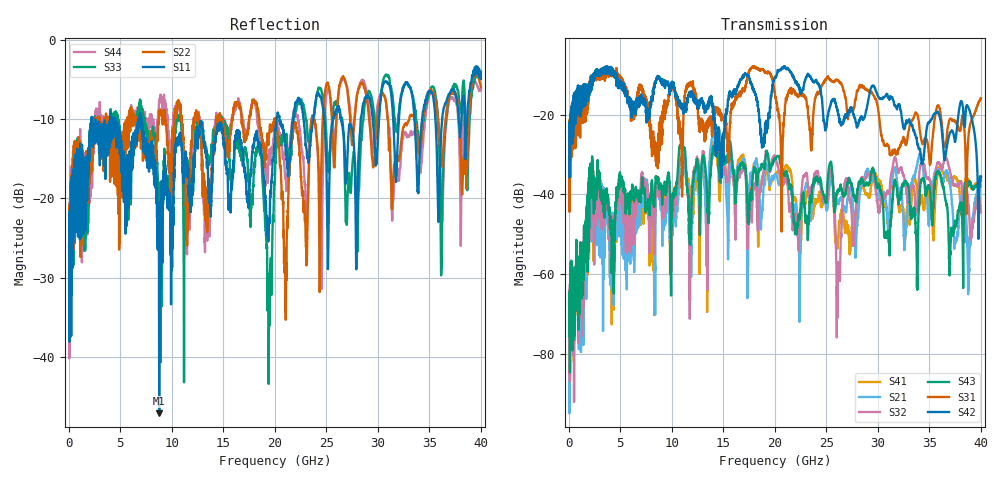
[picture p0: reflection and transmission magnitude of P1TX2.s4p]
!Agilent Technologies,N5245A,MY49151084,A.09.20.08
!Agilent N5245A: A.09.20.08
!Date: Thursday, March 01, 2012 13:18:28
!Correction: S11(Full 4 Port(1,2,3,4))
!S12(Full 4 Port(1,2,3,4))
!S13(Full 4 Port(1,2,3,4))
!S14(Full 4 Port(1,2,3,4))
!S21(Full 4 Port(1,2,3,4))
!S22(Full 4 Port(1,2,3,4))
!S23(Full 4 Port(1,2,3,4))
!S24(Full 4 Port(1,2,3,4))
!S31(Full 4 Port(1,2,3,4))
!S32(Full 4 Port(1,2,3,4))
!S33(Full 4 Port(1,2,3,4))
!S34(Full 4 Port(1,2,3,4))
!S41(Full 4 Port(1,2,3,4))
!S42(Full 4 Port(1,2,3,4))
!S43(Full 4 Port(1,2,3,4))
!S44(Full 4 Port(1,2,3,4))
!S4P File: Measurements: <S11,S12,S13,S14>,
!<S21,S22,S23,S24>,
!<S31,S32,S33,S34>,
!<S41,S42,S43,S44>:
# Hz S  dB  R 50
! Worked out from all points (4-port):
!   3996 points, 50 MHz to 40 GHz, reference 50 ohm
!   strongest paths, dB at 50 MHz, 10.04 GHz, 20.03 GHz, 30.02 GHz, 40 GHz:
!     S42: -24.5, -12.6, -10.8, -15.4, -35.8
!     S31: -25.5, -12.9, -15.1, -18.3, -15.9
!     S43: -67.0, -44.3, -31.1, -37.6, -36.4
!     S32: -64.1, -48.6, -30.6, -43.5, -44.5
!     S21: -69.5, -48.2, -35.1, -38.4, -37.9
!     S41: -64.8, -41.7, -35.2, -36.3, -35.7
!   lowest |S11| = -47.1 dB at 8.79 GHz (marker M1), VSWR 1.01, Z = 49.7 + j0.265 ohm
!   |S11| at or under -10 dB: start of sweep to 2.234 GHz; 4.58 GHz to 6.79 GHz (2.21 GHz wide, 38.9 % of centre); 7.032 GHz to 20.17 GHz (13.13 GHz wide, 96.6 % of centre)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
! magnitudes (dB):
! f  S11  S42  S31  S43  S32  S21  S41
! 50 MHz  -24.1  -24.5  -25.5  -67.0  -64.1  -69.5  -64.8
! 2.18 GHz  -11.9  -11.5  -10.8  -40.8  -45.9  -42.2  -39.3
! 8.79 GHz  -47.1  -10.9  -22.9  -38.7  -39.1  -39.6  -38.4
! 21.03 GHz  -13.1  -8.3  -17.4  -34.5  -36.4  -35.3  -33.1
! 26.17 GHz  -8.4  -19.9  -11.6  -39.0  -57.5  -42.2  -50.4
! 26.92 GHz  -17.7  -20.2  -16.6  -38.9  -36.1  -44.5  -47.2
! 40 GHz  -4.9  -35.8  -15.9  -36.4  -44.5  -37.9  -35.7
